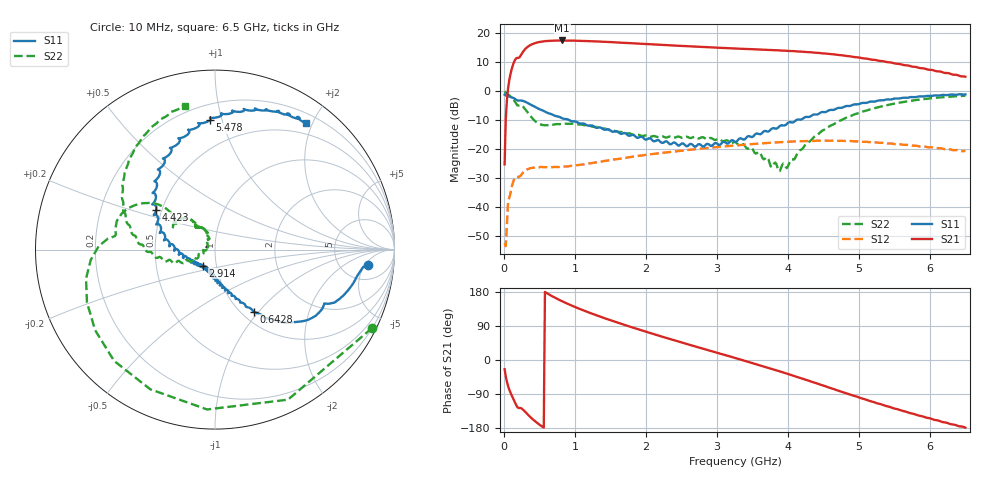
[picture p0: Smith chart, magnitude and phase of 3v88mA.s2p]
!Agilent Technologies,N5230A,MY45000233,A.04.83
!Agilent N5230A: A.04.83
!Date: Friday, August 18, 2006 03:09:24
!Correction: S11(Full 2 Port SOLT,1,2) S21(Full 2 Port SOLT,1,2) S12(Full 2 Port SOLT,1,2) S22(Full 2 Port SOLT,1,2)
!S2P File: Measurements: S11, S21, S12, S22:
# Hz S  dB  R 50
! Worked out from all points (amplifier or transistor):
!   401 points, 10 MHz to 6.5 GHz, reference 50 ohm
!   highest |S21| = 17.3 dB at 821.2 MHz (marker M1)
!   |S21| within 3 dB of that: 298.4 MHz to 3.494 GHz (3.196 GHz wide, 169 % of centre)
!   unconditionally stable (mu >= 1): start of sweep to end of sweep
!   at 1.081 GHz: K = 1.28, MAG = 18.1 dB, |S12| = -25.4 dB
!   at 3.255 GHz: K = 1.08, MAG = 15.0 dB, |S12| = -18.8 dB
!   at 6.5 GHz: K = 1.04, MAG = 11.6 dB, |S12| = -20.8 dB
!   S11 on the Smith chart (normalised r, x): 10 MHz: 9, -6; 642.8 MHz: 1.13, -0.94; 2.914 GHz: 0.86, -0.16; 4.423 GHz: 0.47, +0.24; 5.478 GHz: 0.30, +0.92; 6.5 GHz: 0.33, +1.91
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1e7  -1.34 -5.8  -25.32 -24.3  -52.47 1.0  -0.19 -26.6
7.49e7  -1.99 -13.1  3.53 -77.8  -36.76 130.2  -1.55 -132.2
1.398e8  -2.55 -21.7  9.73 -105.2  -30.67 85.5  -3.17 -175.3
3.0205e8  -3.77 -37.3  14.40 -137.1  -27.42 48.6  -6.39 147.4
4.643e8  -5.88 -50.0  16.58 -165.4  -26.30 27.4  -10.93 141.9
6.42775e8  -7.79 -58.1  17.18 172.2  -26.25 16.5  -11.76 151.6
8.2125e8  -9.46 -62.2  17.30 154.9  -26.09 12.1  -11.37 149.7
1.097075e9  -11.24 -70.3  17.17 132.5  -25.37 7.4  -11.63 139.4
1.324225e9  -12.69 -76.2  16.95 116.5  -24.52 2.8  -12.54 132.2
1.5676e9  -13.94 -82.6  16.66 100.7  -23.57 -3.2  -13.84 127.8
2.18415e9  -17.07 -97.7  15.84 64.1  -21.47 -22.1  -15.93 129.7
2.57355e9  -19.10 -112.2  15.35 42.5  -20.39 -35.9  -15.77 129.4
2.914275e9  -18.96 -127.6  14.93 23.9  -19.55 -48.6  -16.22 124.7
3.255e9  -17.58 -145.9  14.54 5.5  -18.81 -62.2  -17.61 118.2
3.822875e9  -13.01 -179.0  13.94 -26.4  -17.76 -87.0  -24.67 139.9
4.342075e9  -8.39 149.4  13.18 -57.9  -17.23 -112.4  -16.51 -153.5
4.4232e9  -8.06 145.9  13.05 -62.8  -17.16 -116.4  -15.01 -158.5
4.8775e9  -5.19 122.0  11.86 -91.2  -17.26 -139.5  -8.77 -178.0
5.42915e9  -2.99 96.9  9.78 -123.4  -18.10 -166.1  -4.74 152.2
5.477825e9  -2.83 92.2  9.59 -126.9  -18.19 -169.0  -4.53 150.8
5.932125e9  -1.86 74.1  7.60 -151.2  -19.18 170.8  -2.81 127.7
6.5e9  -1.22 54.2  4.84 -178.6  -20.78 147.8  -1.72 101.9
